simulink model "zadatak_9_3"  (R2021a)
settings: Solver=VariableStepAuto  StartTime=0.0  StopTime=50  RelTol=1e-3

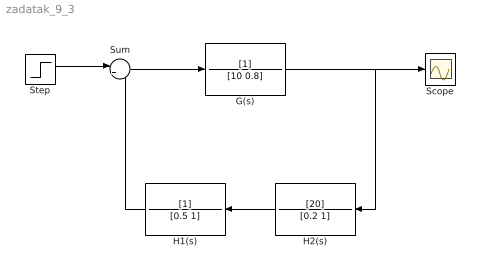
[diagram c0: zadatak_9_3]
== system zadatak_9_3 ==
  G(s) : TransferFcn  Denominator=[10 0.8]
  H1(s) : TransferFcn  Denominator=[0.5 1]
  H2(s) : TransferFcn  Numerator=[20]  Denominator=[0.2 1]
  Scope : Scope
  Step : Step  Time=10  After=50  SampleTime=0
  Sum : Sum  Inputs=|+-
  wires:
  H2(s)/1 -> H1(s)/1
  G(s)/1 -> Scope/1, H2(s)/1
  H1(s)/1 -> Sum/2
  Sum/1 -> G(s)/1
  Step/1 -> Sum/1
